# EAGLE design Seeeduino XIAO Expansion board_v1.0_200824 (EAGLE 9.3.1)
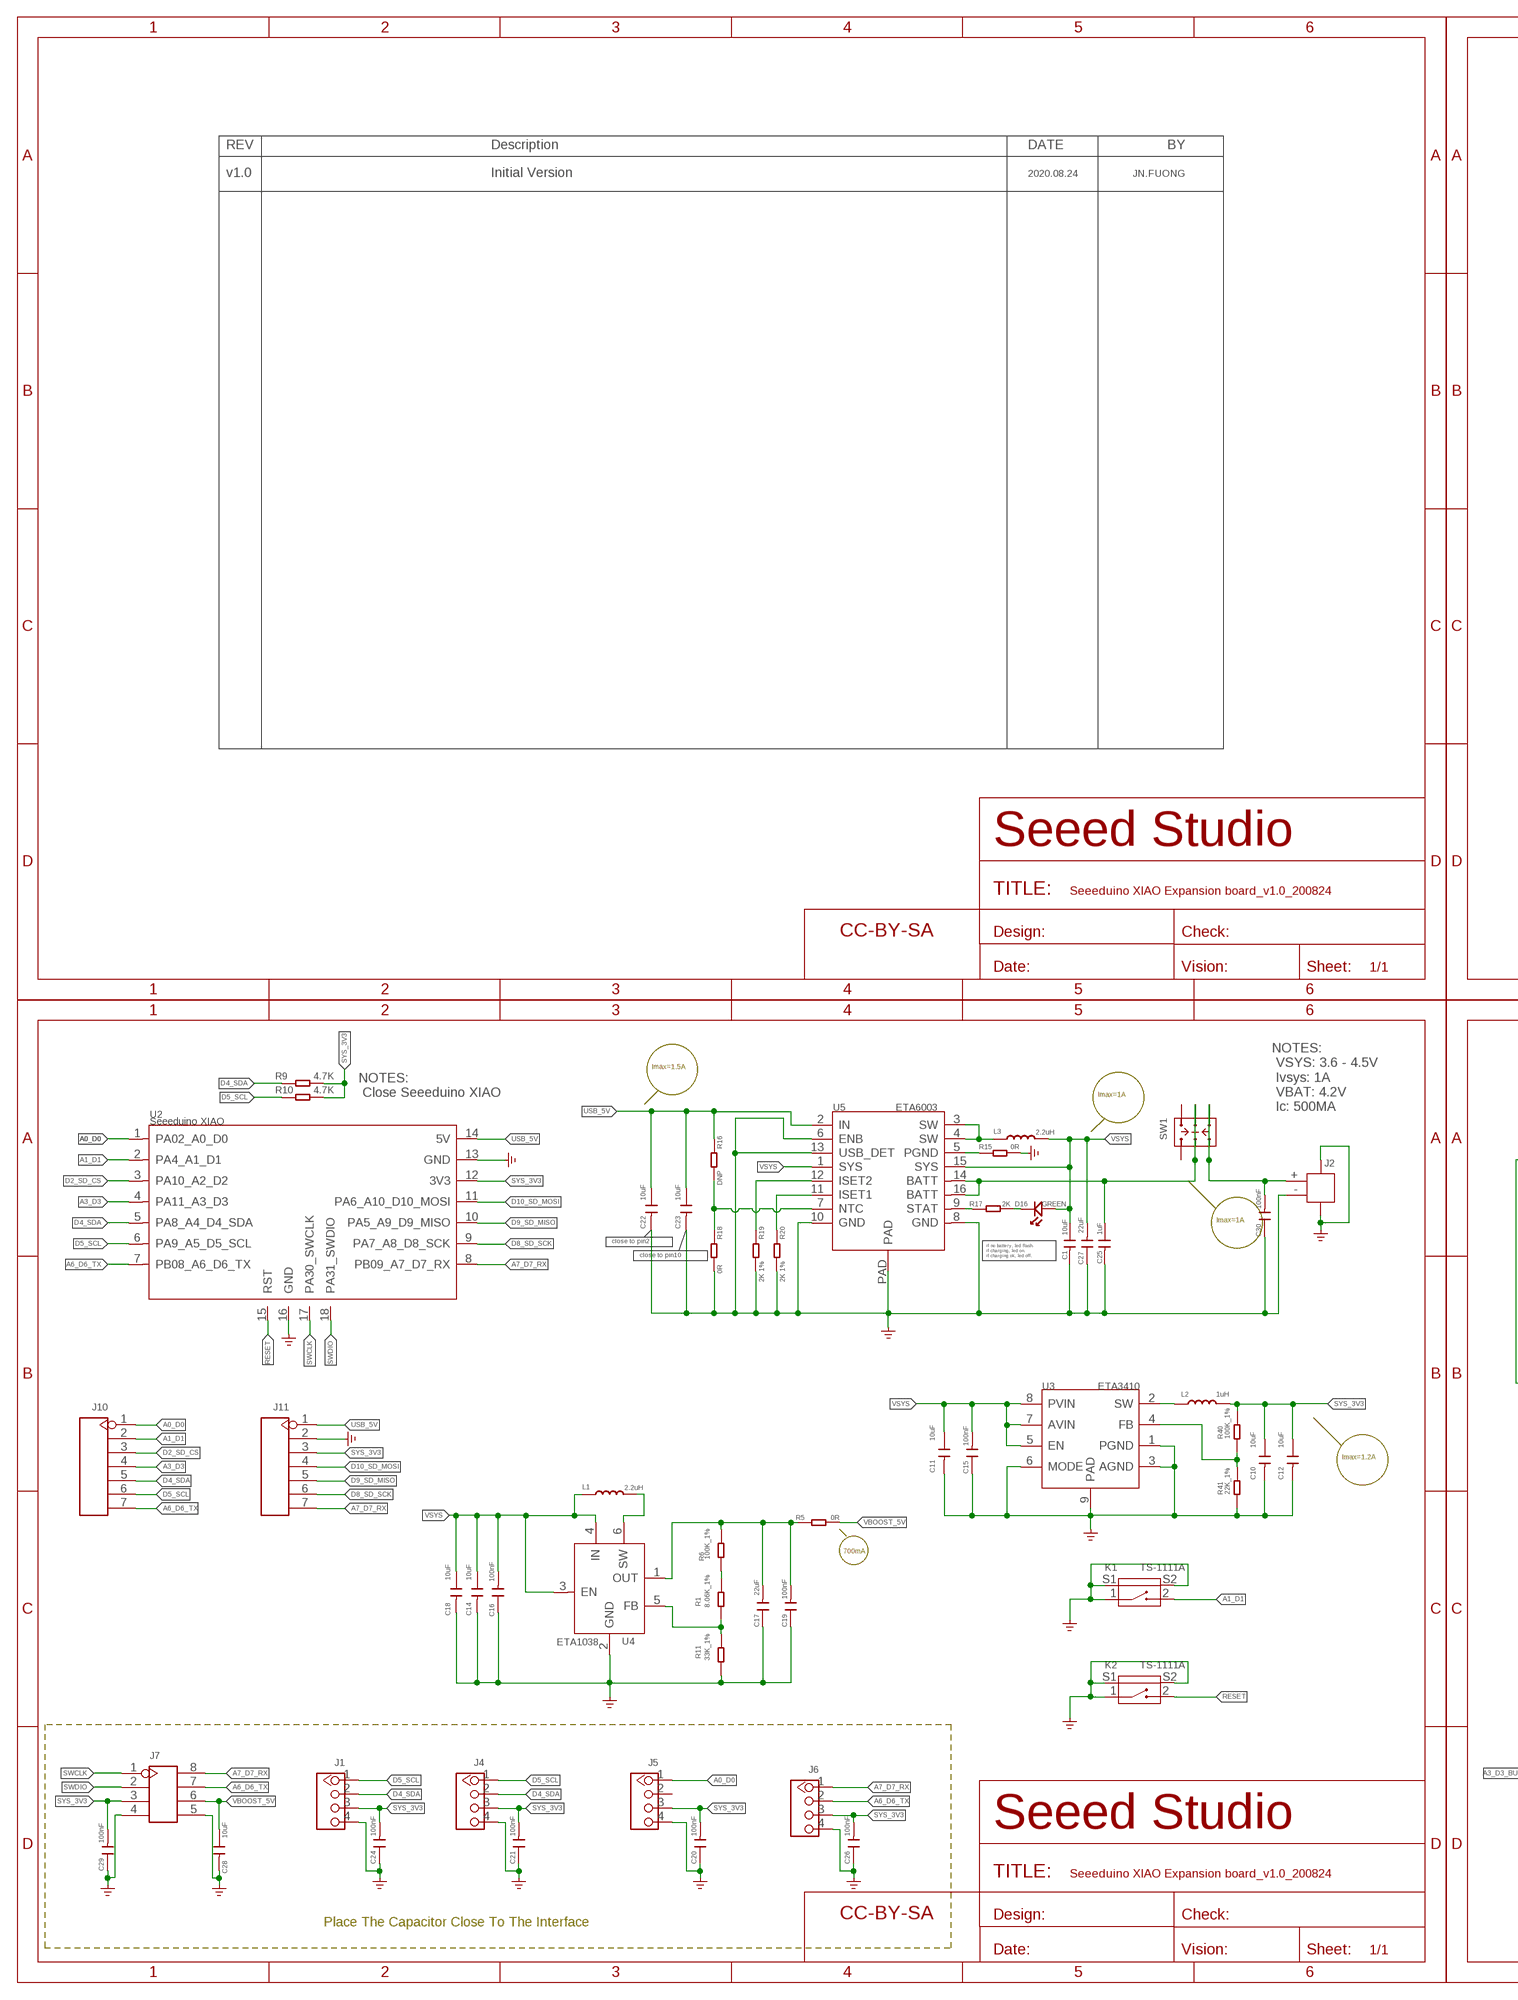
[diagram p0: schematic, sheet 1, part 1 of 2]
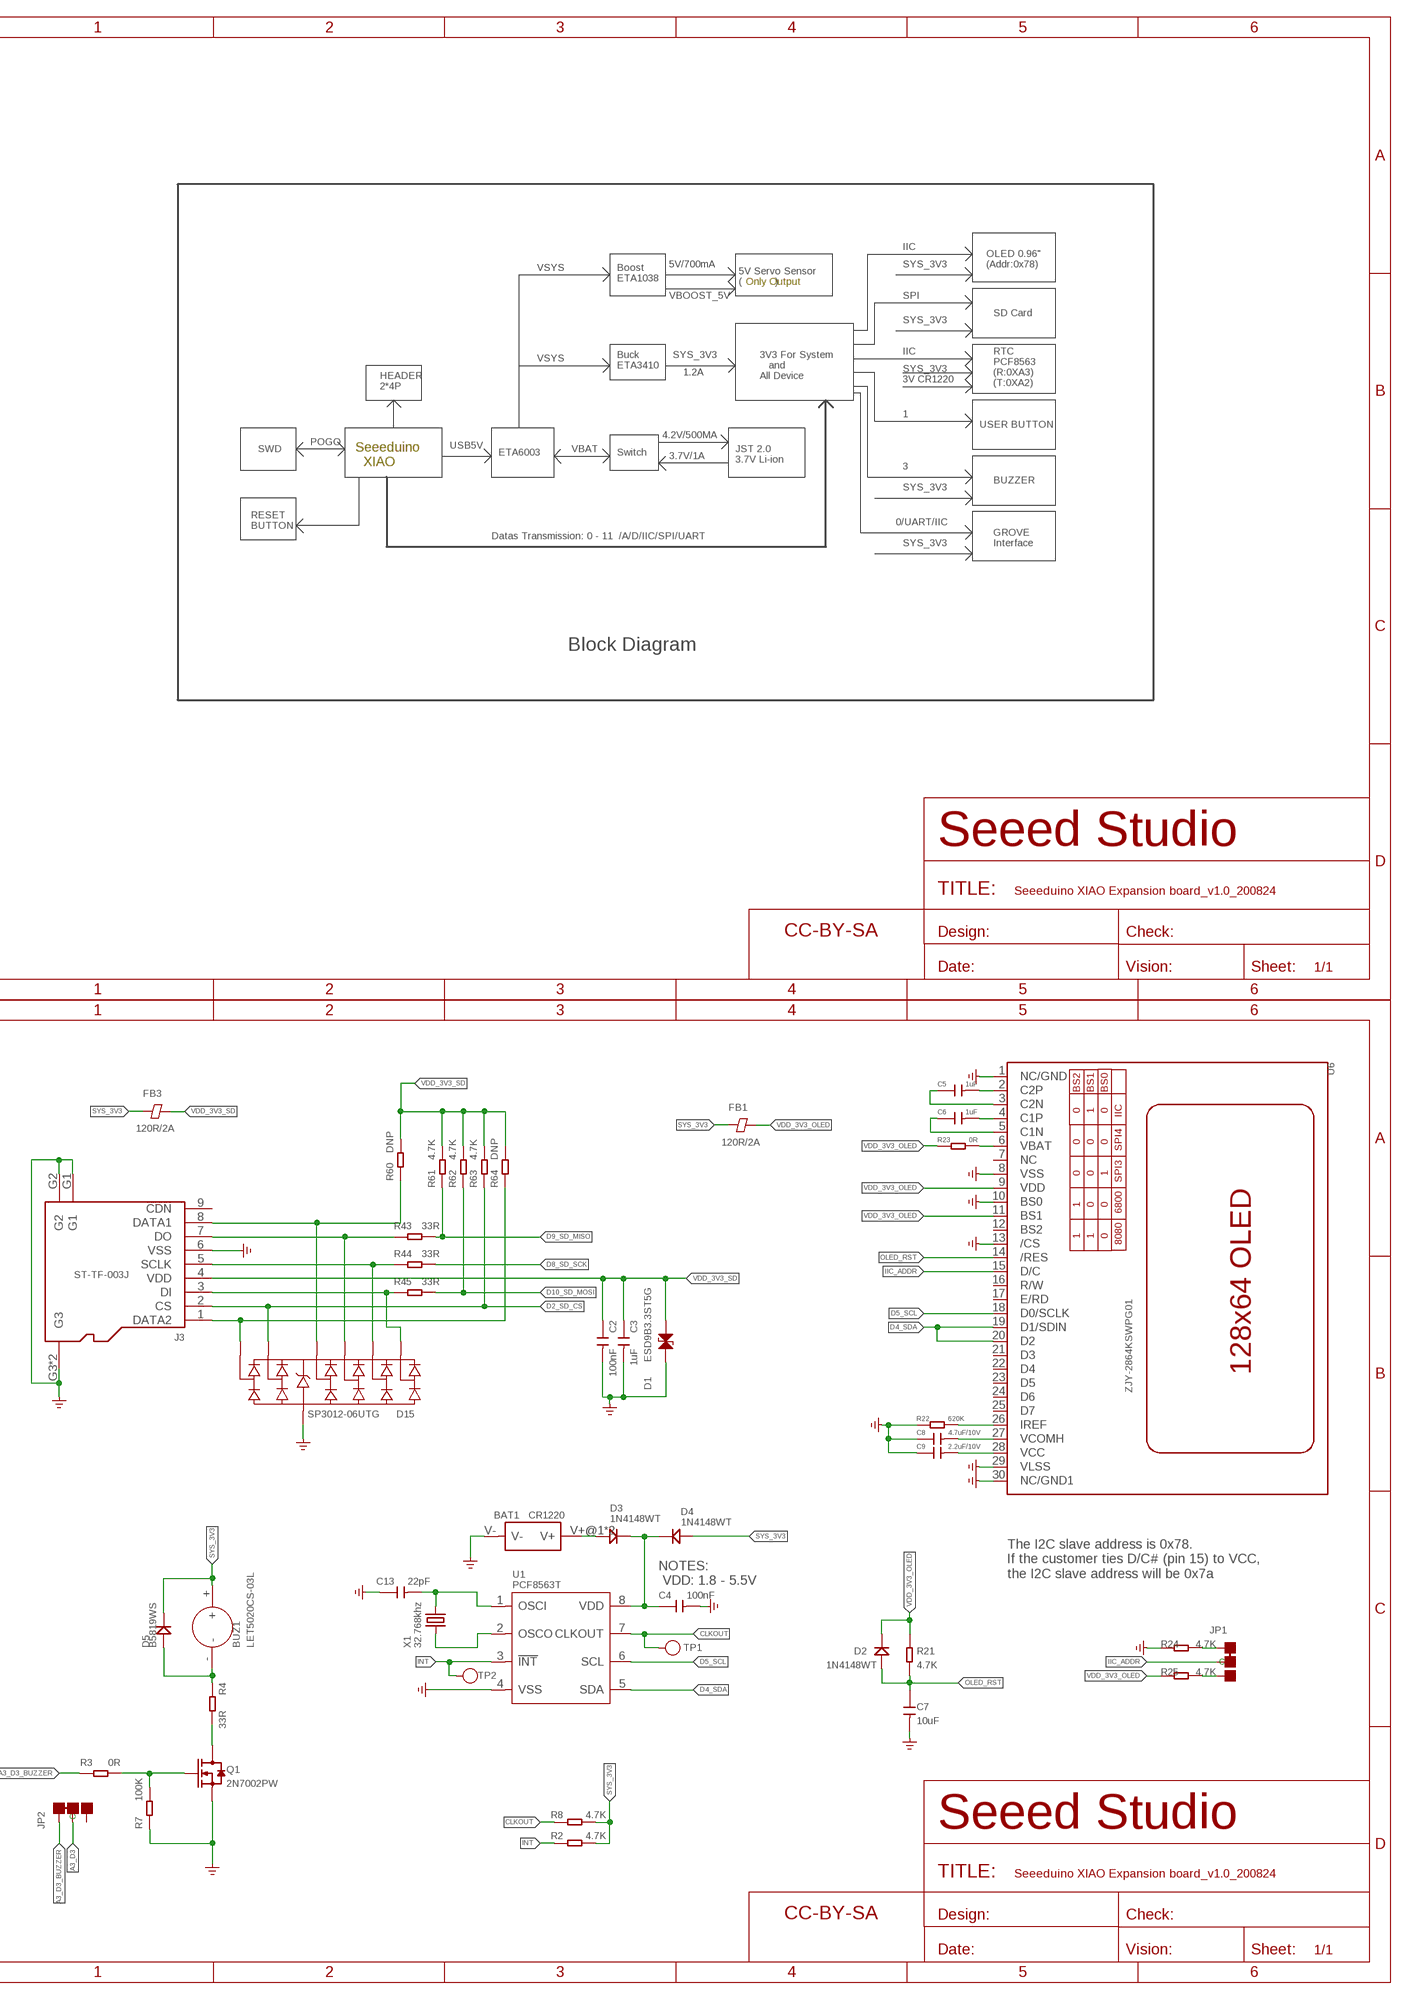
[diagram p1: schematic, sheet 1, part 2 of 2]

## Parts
BAT1  CR1220  BAT-HOLDER-KST-1206  [BAT2P-SMD-13.2X12.1X3.2MM]
BUZ1  LET5020CS-03L  BUZZER-312020004  [BZ3-SMD-5.0X5.0X2.5MM]
C1  10uF  C-0603  [C0603]
C2  100nF  C-0402  [C0402]
C3  1uF  C-0402  [C0402]
C4  100nF  C-0402  [C0402]
C5  1uF  C-0402  [C0402]
C6  1uF  C-0402  [C0402]
C7  10uF  C-0603  [C0603]
C8  4.7uF/10V  C-0603  [C0603]
C9  2.2uF/10V  C-0603  [C0603]
C10  10uF  C-0603  [C0603]
C11  10uF  C-0603  [C0603]
C12  10uF  C-0603  [C0603]
C13  22pF  C-0402  [C0402]
C14  10uF  C-0603  [C0603]
C15  100nF  C-0402  [C0402]
C16  100nF  C-0402  [C0402]
C17  22uF  C-0603  [C0603]
C18  10uF  C-0603  [C0603]
C19  100nF  C-0402  [C0402]
C20  100nF  C-0402  [C0402]
C21  100nF  C-0402  [C0402]
C22  10uF  C-0603  [C0603]
C23  10uF  C-0603  [C0603]
C24  100nF  C-0402  [C0402]
C25  1uF  C-0402  [C0402]
C26  100nF  C-0402  [C0402]
C27  22uF  C-0603  [C0603]
C28  10uF  C-0603  [C0603]
C29  100nF  C-0402  [C0402]
C30  100nF  C-0603  [C0603]
D1  ESD9B3.3ST5G  D-ESD-2P-DOUBLE-0402  [ESD-0402]
D2  1N4148WT  DIODE'0603'  [SOD-523]
D3  1N4148WT  DIODE'0603'  [SOD-523]
D4  1N4148WT  DIODE'0603'  [SOD-523]
D5  B5819WS  DIODE'0805'  [SOD-323]
D15  SP3012-06UTG  D-ESD-14P  [UDFN14-0.5-3.5X1.35X0.5MM]
D16  GREEN  LED-0402  [LED-0402]
FB1  120R/2A  FERRITE-BEAD-0402  [F0402]
FB3  120R/2A  FERRITE-BEAD-0402  [F0402]
FR1  SEEEDSTUDIO-OPEN-SCH-FRAME  [SEEEDSTUDIO-PCB-FRAME]
FR2  SEEEDSTUDIO-OPEN-SCH-FRAME  [SEEEDSTUDIO-PCB-FRAME]
FR3  SEEEDSTUDIO-OPEN-SCH-FRAME  [SEEEDSTUDIO-PCB-FRAME]
FR5  SEEEDSTUDIO-OPEN-SCH-FRAME  [SEEEDSTUDIO-PCB-FRAME]
J1  GROVE-CONNECTOR-DIP-320110034  [HW4-2.0-90D]
J2  JST-2P-SMD'2.0'  [HW2-SMD-2.0-90D]
J3  ST-TF-003J  MICRO-SD-CARD-HOLDER-9P-320090000  [MICRO-SD9+4P-SMD-16.1X14.5X1.85MM]
J4  GROVE-CONNECTOR-DIP-320110034  [HW4-2.0-90D]
J5  GROVE-CONNECTOR-DIP-320110034  [HW4-2.0-90D]
J6  GROVE-CONNECTOR-DIP-320110034  [HW4-2.0-90D]
J7  HEADER-2X4P-2.54-SMD  [H2X4-SMD-2.54]
J10  HEADER-7P-2.54  [H7-2.54]
J11  HEADER-7P-2.54  [H7-2.54]
JP1  JP-3P-SHORT  [3P-SMD-SHORT]
JP2  JP-3P-SHORT  [3P-SMD-SHORT]
K1  TS-1111A  BUTTON-2+2P'HQ-TP-1100A'  [SW4-SMD-4.5X3.8X1.8MM-90D]
K2  TS-1111A  BUTTON-2+2P'HQ-TP-1100A'  [SW4-SMD-4.5X3.8X1.8MM-90D]
L1  2.2uH  INDUCTOR/FERRITE-BEAD'0806'  [L0806]
L2  1uH  L-MPM201610SR33_T  [L201610]
L3  2.2uH  INDUCTOR/FERRITE-BEAD'0806'  [L0806]
Q1  2N7002PW  MOSFET-N-SI1304BDL  [SOT-323]
R1  8.06K_1%  R-0402  [R0402]
R2  4.7K  R-0402  [R0402]
R3  0R  R-0402  [R0402]
R4  33R  R-0402  [R0402]
R5  0R  R-0603  [R0603]
R6  100K_1%  R-0402  [R0402]
R7  100K  R-0402  [R0402]
R8  4.7K  R-0402  [R0402]
R9  4.7K  R-0402  [R0402]
R10  4.7K  R-0402  [R0402]
R11  33K_1%  R-0402  [R0402]
R15  0R  R-0402  [R0402]
R16  DNP  R-0402  [R0402]
R17  2K  R-0402  [R0402]
R18  0R  R-0402  [R0402]
R19  2K 1%  R-0402  [R0402]
R20  2K 1%  R-0402  [R0402]
R21  4.7K  R-0402  [R0402]
R22  620K  R-0402  [R0402]
R23  0R  R-0402  [R0402]
R24  4.7K  R-0402  [R0402]
R25  4.7K  R-0402  [R0402]
R40  100K_1%  R-0402  [R0402]
R41  22K_1%  R-0402  [R0402]
R43  33R  R-0402  [R0402]
R44  33R  R-0402  [R0402]
R45  33R  R-0402  [R0402]
R60  DNP  R-0402  [R0402]
R61  4.7K  R-0402  [R0402]
R62  4.7K  R-0402  [R0402]
R63  4.7K  R-0402  [R0402]
R64  DNP  R-0402  [R0402]
SW1  SWITCH-2CH-6P-311030004  [SW6-2.54-9.0X3.5X3.2MM-90D]
TP1  TEST-POINT'4545'  [TP-D45MIL]
TP2  TEST-POINT'4545'  [TP-D45MIL]
U1  PCF8563T  RTC-PCF8563T  [SOP8-1.27-5X3.9MM]
U2  Seeeduino XIAO  MOUDLE-SEEEDUINO-XIAO-TEST-DIP  [MOUDLE14P-2.54-21X17.8MM-TEST]
U3  ETA3410  CONVERTER-ETA3410  [DFN8G-0.5-2X2MM]
U4  ETA1038  CONVERTER-ETA1038  [SOT-23-6]
U5  ETA6003  PMIC-ETA6003-310990023  [QFN16GA-0.5-3X3MM]
U6  ZJY-2864KSWPG01  OLED-12864-30P  [OLED30P-0.7-24.74X16.9MM]
X1  32.768khz  CRYSTAL-2P'NX2012SA'  [X2-SMD-L2.0X1.2X0.55MM]

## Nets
A0_D0: J5.1 J10.1 U2.1(PA02_A0_D0)
A1_D1: J10.2 K1.2 U2.2(PA4_A1_D1)
A3_D3: J10.4 JP2.MM(C) U2.4(PA11_A3_D3)
A3_D3_BUZZER: JP2.11(L) R3.1
A6_D6_TX: J6.2 J7.7 J10.7 U2.7(PB08_A6_D6_TX)
A7_D7_RX: J6.1 J7.8 J11.7 U2.8(PB09_A7_D7_RX)
CLKOUT: R8.1 TP1.T U1.7(CLKOUT)
D2_SD_CS: D15.6 D15.9 J3.2(CS) J10.3 R63.1 U2.3(PA10_A2_D2)
D4_SDA: J1.2 J4.2 J10.5 R9.1 U1.5(SDA) U2.5(PA8_A4_D4_SDA) U6.19(D1/SDIN) U6.20(D2)
D5_SCL: J1.1 J4.1 J10.6 R10.1 U1.6(SCL) U2.6(PA9_A5_D5_SCL) U6.18(D0/SCLK)
D8_SD_SCK: J11.6 R44.2 U2.9(PA7_A8_D8_SCK)
D9_SD_MISO: J11.5 R43.2 R61.1 U2.10(PA5_A9_D9_MISO)
D10_SD_MOSI: J11.4 R45.2 R62.1 U2.11(PA6_A10_D10_MOSI)
E_VBAT: C30.2 J2.+ SW1.CH1B SW1.CH2B
GND: BAT1.V- C1.2 C2.2 C3.2 C4.2 C7.2 C8.1 C9.1 C10.2 C11.2 C12.2 C13.1 C14.2 C15.1 C16.1 C17.1 C18.2 C19.1 C20.1 C21.1 C22.2 C23.2 C24.1 C25.2 C26.1 C27.1 C28.2 C29.1 C30.1 D1.1 D15.5 D15.10 J1.4 J2.3 J2.4 J2.- J3.6(VSS) J3.G1 J3.G2 J3.G3 J3.G4(G3) J4.4 J5.4 J6.4 J7.4 J7.5 J11.2 K1.1 K1.S1 K1.S2 K2.1 K2.S1 K2.S2 Q1.2(S) R7.1 R11.2 R15.2 R18.2 R19.2 R20.2 R22.2 R24.1 R41.1 U1.4(VSS) U2.13(GND) U2.16(GND) U3.1(PGND) U3.3(AGND) U3.6(MODE) U3.9(PAD) U4.2(GND) U5.6(ENB) U5.8(GND) U5.10(GND) U5.13(USB_DET) U5.PAD U6.1(NC/GND) U6.8(VSS) U6.10(BS0) U6.13(/CS) U6.29(VLSS) U6.30(NC/GND1) ; supply symbol labelled GND_POWER
IIC_ADDR: JP1.MM(C) U6.15(D/C)
INT: R2.1 TP2.T U1.3(!INT)
N$1: L1.2 U4.6(SW)
N$5: BAT1.V+@1(V+) BAT1.V+@2(V+) D3.+
N$6: Q1.3(D) R4.2
N$7: BUZ1.- D5.+ R4.1
N$8: Q1.1(G) R3.2 R7.2
N$9: C5.2 U6.2(C2P)
N$10: C13.2 U1.1(OSCI) X1.2
N$11: U1.2(OSCO) X1.1
N$12: C6.2 U6.4(C1P)
N$13: C5.1 U6.3(C2N)
N$14: C6.1 U6.5(C1N)
N$15: R22.1 U6.26(IREF)
N$16: C8.2 U6.27(VCOMH)
N$17: C9.2 U6.28(VCC)
N$18: R23.2 U6.6(VBAT)
N$19: JP1.11(L) R24.2
N$20: JP1.00(R) R25.2
N$21: R40.1 R41.2 U3.4(FB)
N$22: C17.2 C19.2 R5.2 R6.1 U4.1(OUT)
N$23: C4.1 D3.- D4.- U1.8(VDD)
N$24: R1.1 R6.2
N$26: L3.1 U5.3(SW) U5.4(SW)
N$27: R1.2 R11.1 U4.5(FB)
N$29: L2.1 U3.2(SW)
N$30: D16.- R17.1
N$31: R17.2 U5.9(STAT)
N$33: R16.2 R18.1 U5.7(NTC)
N$34: R20.1 U5.11(ISET1)
N$36: R19.1 U5.12(ISET2)
N$37: R15.1 U5.5(PGND)
N$64: D15.1 D15.14 J3.8(DATA1) R60.1
N$72: D15.7 D15.8 J3.1(DATA2) R64.1
N$76: D15.2 D15.13 J3.7(DO) R43.1
N$77: D15.3 D15.12 J3.5(SCLK) R44.1
N$78: D15.4 D15.11 J3.3(DI) R45.1
OLED_RST: C7.1 D2.+ R21.1 U6.14(/RES)
RESET: K2.2 U2.15(RST)
SWCLK: J7.1 U2.17(PA30_SWCLK)
SWDIO: J7.2 U2.18(PA31_SWDIO)
SYS_3V3: BUZ1.+ C10.1 C12.1 C20.2 C21.2 C24.2 C26.2 C29.2 D4.+ D5.- FB1.1 FB3.1 J1.3 J4.3 J5.3 J6.3 J7.3 J11.3 L2.2 R2.2 R8.2 R9.2 R10.2 R40.2 U2.12(3V3)
USB_5V: C22.1 C23.1 J11.1 R16.1 U2.14(5V) U5.2(IN)
VBAT: C25.1 SW1.COM1 SW1.COM2 U5.14(BATT) U5.16(BATT)
VBOOST_5V: C28.1 J7.6 R5.1
VDD_3V3_OLED: D2.- FB1.2 R21.2 R23.1 R25.1 U6.9(VDD) U6.11(BS1)
VDD_3V3_SD: C2.1 C3.1 D1.2 FB3.2 J3.4(VDD) R60.2 R61.2 R62.2 R63.2 R64.2
VSYS: C1.1 C11.1 C14.1 C15.2 C16.2 C18.1 C27.2 D16.+ L1.1 L3.2 U3.5(EN) U3.7(AVIN) U3.8(PVIN) U4.3(EN) U4.4(IN) U5.1(SYS) U5.15(SYS)
Unconnected: J3.9(CDN) J5.2 JP2.00(R) SW1.CH1A SW1.CH2A U6.7(NC) U6.12(BS2) U6.16(R/W) U6.17(E/RD) U6.21(D3) U6.22(D4) U6.23(D5) U6.24(D6) U6.25(D7)

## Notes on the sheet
- v1.0 | Initial Version | 2020.08.24 | JN.FUONG
- IIC
- VSYS
- 5V/700mA | SYS_3V3
- OLED 0.96"
  (Addr:0x78)
- Boost
  ETA1038
- 5V Servo Sensor
  (           )
- Only Output
- VBOOST_5V | SPI
- SD Card
- SYS_3V3
- VSYS | IIC
- SYS_3V3
- Buck
  ETA3410
- SYS_3V3
- 1.2A
- 3V3 For System 
     and 
  All Device
- 3V CR1220
- RTC
  PCF8563
  (R:0XA3)
  (T:0XA2)
- HEADER
  2*4P
- 1
- USER BUTTON
- 4.2V/500MA
- POGO
- USB5V
- SWD | VBAT
- ETA6003 | Switch
- 3.7V/1A
- JST 2.0
  3.7V Li-ion
- Seeeduino
    XIAO
- 3
- BUZZER
- SYS_3V3
- 0/UART/IIC
- RESET
  BUTTON
- Datas Transmission: 0 - 11  /A/D/IIC/SPI/UART
- SYS_3V3
- GROVE 
  Interface
- Block Diagram
- Imax=1.5A
- NOTES:
   Close Seeeduino XIAO
- Imax=1A
- NOTES:
   VSYS: 3.6 - 4.5V
   Ivsys: 1A
   VBAT: 4.2V
   Ic: 500MA
- Imax=1A
- close to pin2
- close to pin10
- if no battery, led flash.
  if charging, led on.
  if charging ok, led off.
- Imax=1.2A
- 700mA
- The I2C slave address is 0x78.
  If the customer ties D/C# (pin 15) to VCC,
  the I2C slave address will be 0x7a
- NOTES:
   VDD: 1.8 - 5.5V
- Place The Capacitor Close To The Interface

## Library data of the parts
BAT1 = Connector-new:BAT-HOLDER: BAT2P-13.5-CR1220:320170002;BAT2P-SMD-20.5-CR1632:320170007;METAL-CR2032-D20.0*H6.3MM:320170003;METAL-CR2032-SMD:320170006;PLASTIC-CR1220-L15.06*W13.0*H4.1MM:32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
BUZ1 = Discrete-new:BUZZER
C1-C30 = Discrete-small:C*: Ceramic Capacitors
D1 = Discrete-small:D-ESD-2P-DOUBLE
D2-D5 = Discrete-new:DIODE
D15 = Discrete-new:D-ESD-14P
D16 = Discrete-small:LED
FB1 FB3 = Discrete-new:FERRITE-BEAD
FR1-FR3 FR5 = moudle-new:SEEEDSTUDIO-OPEN-SCH-FRAME
J1 J4-J6 = Connector-new:GROVE-CONNECTOR-DIP
J2 = Connector-new:JST-2P-SMD
J3 = Connector-new:MICRO-SD-CARD-HOLDER-9P; SKU: 320090000
J7 = Connector-new:HEADER-2X4P
J10 J11 = Connector-new:HEADER-7P
JP1 JP2 = Discrete-new:JP-3P-SHORT
K1 K2 = Discrete-new:BUTTON-2+2P: SW4-SMD-4.5X3.8X1.8MM-90D:311020035;SW4-SMD-7.0X3.5X3.5MM-90D:311020023
L1 L3 = Discrete-new:INDUCTOR/FERRITE-BEAD
L2 = Discrete-new:L
Q1 = Discrete-new:MOSFET-N: IRLL014: http://www.vishay.com/docs/91319/sihll014.pdf
R1-R11 R15-R25 R40 R41 R43-R45 R60-R64 = Discrete-small:R*
SW1 = Switch:SWITCH-2CH-6P
TP1 TP2 = Discrete-new:TEST-POINT; PARTNO: DNP
U1 = IC-new:RTC-PCF8563T
U2 = moudle-new:MOUDLE-SEEEDUINO-XIAO-TEST
U3 = IC-new:CONVERTER-ETA3410: 3MHZ 2A High Step-Down Converter in DFN2x2-8L Package
U4 = IC-new:CONVERTER-ETA1038
U5 = IC-new:PMIC-ETA6003
U6 = moudle-new:OLED-128*64-30P: 308020008
X1 = Discrete-new:CRYSTAL-2P

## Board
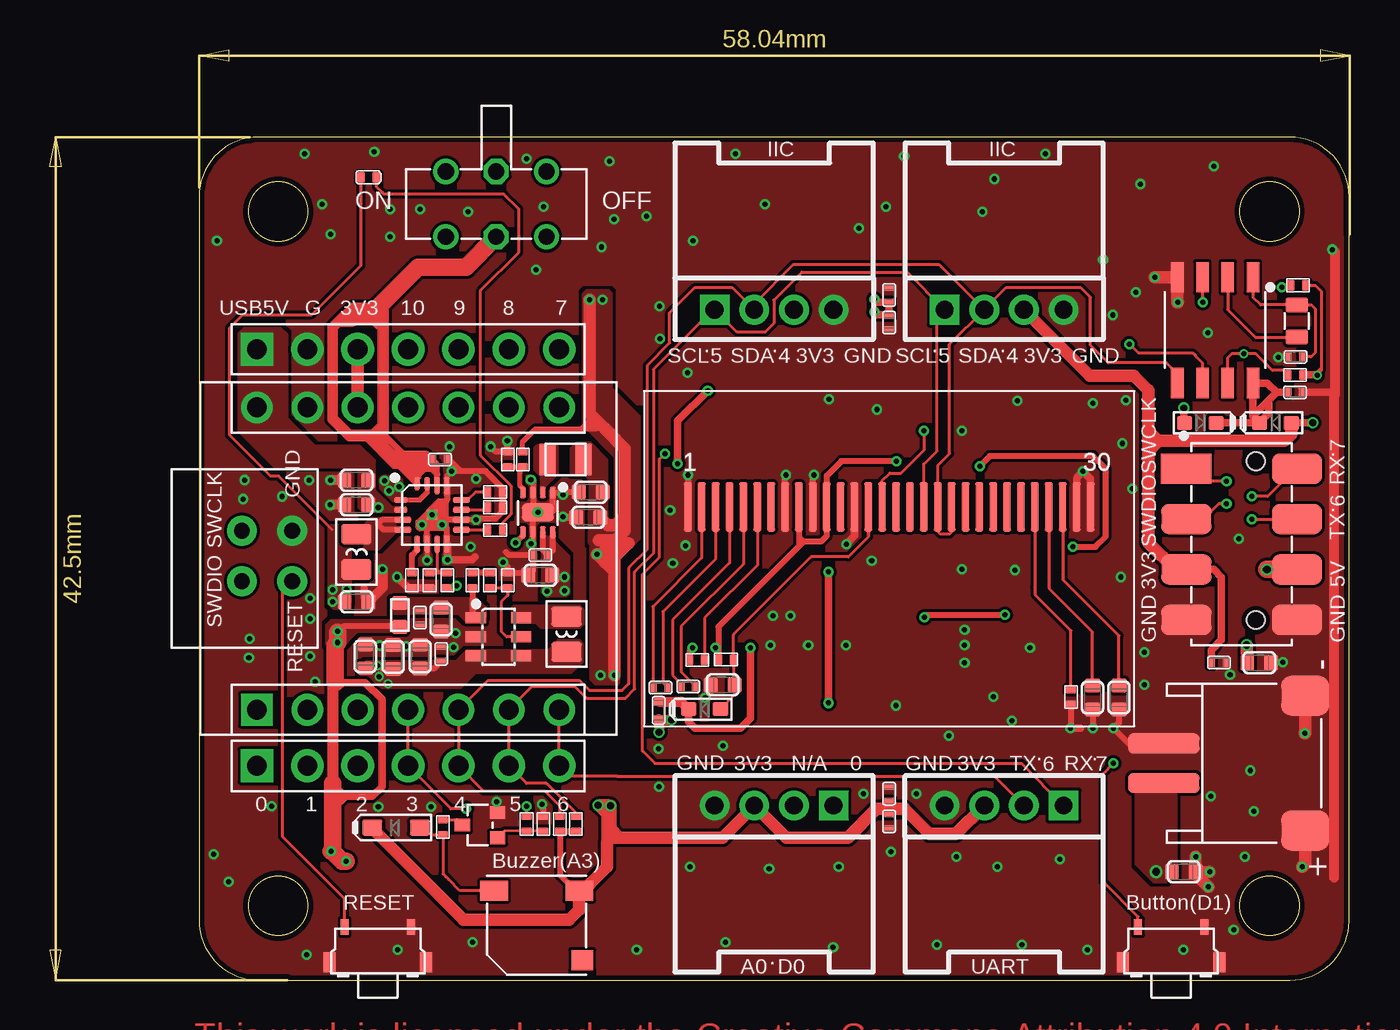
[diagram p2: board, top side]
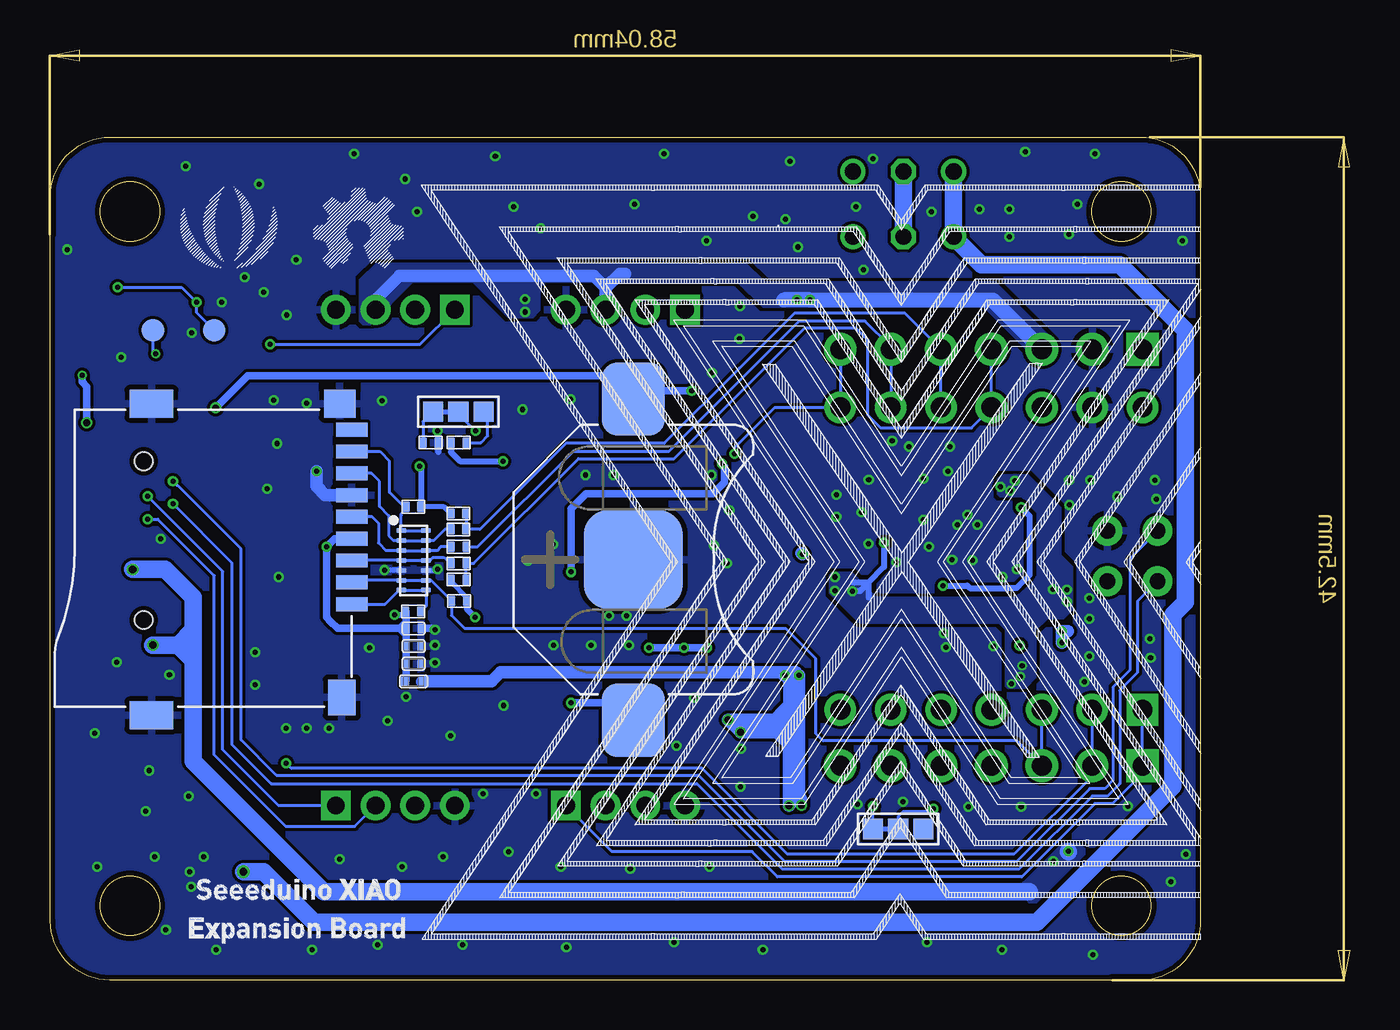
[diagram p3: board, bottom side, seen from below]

Size 65.58 x 46.91 mm. Coordinates in mm from the lower left corner, seen from the top.
Outline: 62.54,42.5 10.54,42.5 arc90 7.54,39.5 7.54,3 arc90 10.54,0 62.54,0 arc90 65.54,3 65.54,39.5 arc90 62.54,42.5
Outline: circle at 11.53,38.75 radius 1.5
Outline: circle at 61.53,38.75 radius 1.5
Outline: circle at 61.53,3.75 radius 1.5
Outline: circle at 11.53,3.75 radius 1.5
Copper layers (1*16): Top 0.035mm / dielectric 1.5mm / Bottom 0.035mm
Design rules "SeeedStudio_2layer_DRU_no_angle_20140221": minimum track width 1mil, minimum drill 10mil, track to track 6mil, track to pad 6mil, pad to pad 6mil, via to via 6mil, smd to smd 0mil, copper to edge 10mil, drill to drill 10mil, minimum pad ring 4mil, minimum via ring 4mil, stop-mask expansion 2mil, vias tented up to drill 25mil, thermal gap 10mil

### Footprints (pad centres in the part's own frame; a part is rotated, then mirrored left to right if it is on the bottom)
BAT2P-SMD-13.2X12.1X3.2MM = smd 3.7 x 3.2: V+@1 -8.1,0; V+@2 8.1,0 | smd 5 x 5: V- 0,0
BZ3-SMD-5.0X5.0X2.5MM = smd 1.4 x 1: + -2.15,-1.75; - 2.15,-1.75 | smd 1.1 x 1: NC -2.3,1.75
C0603 = smd 0.762 x 0.696: 1 0,0.602; 2 0,-0.602
C0402 = smd 0.508 x 0.385: 1 0,0.383; 2 0,-0.383
ESD-0402 = smd 0.385 x 0.508: 1 0.383,0; 2 -0.383,0
SOD-523 = smd 0.762 x 0.7: + 0.8,0; - -0.8,0
SOD-323 = smd 1 x 0.8: + 1.2,0; - -1.2,0
UDFN14-0.5-3.5X1.35X0.5MM = smd 0.25 x 0.5: 1 -1.5,-0.625; 2 -1,-0.625; 3 -0.5,-0.625; 4 0,-0.625; 5 0.5,-0.625; 6 1,-0.625; 7 1.5,-0.625; 8 1.5,0.625; 9 1,0.625; 10 0.5,0.625; 11 0,0.625; 12 -0.5,0.625; 13 -1,0.625; 14 -1.5,0.625
LED-0402 = smd 0.385 x 0.508: + -0.383,0; - 0.383,0
F0402 = smd 0.445 x 0.508: 1 -0.445,0; 2 0.445,0
HW4-2.0-90D = drill 0.9 pad 1.5 square: 1 -3,0 | drill 0.9 pad 1.5: 2 -1,0; 3 1,0; 4 3,0
HW2-SMD-2.0-90D = smd 2 x 2.4: 3 3.4,-2.181; 4 -3.4,-2.181 | smd 1 x 3.6: + -1,4.953; - 1,4.953
MICRO-SD9+4P-SMD-16.1X14.5X1.85MM = smd 1.6 x 0.7: 1 0,2.25; 2 0,1.15; 3 0,0.05; 4 0,-1.05; 5 0,-2.15; 6 0,-3.25; 7 0,-4.35; 8 0,-5.45; 9 0,-6.55 | smd 1.6 x 1.4: G1 0.6,-7.85 | smd 2.2 x 1.4: G2 10.1,-7.85; G3 10.1,7.85 | smd 1.4 x 1.8: G4 0.5,6.95 | hole 0.9: 10.5,-4.95; 10.5,3.05
H2X4-SMD-2.54 = smd 2.54 x 1.524: 1 -2.794,3.81; 2 -2.794,1.27; 3 -2.794,-1.27; 4 -2.794,-3.81; 5 2.794,-3.81; 6 2.794,-1.27; 7 2.794,1.27; 8 2.794,3.81
H7-2.54 = drill 1 pad 1.651 square: 1 0,7.62 | drill 1 pad 1.651: 2 0,5.08; 3 0,2.54; 4 0,0; 5 0,-2.54; 6 0,-5.08; 7 0,-7.62
3P-SMD-SHORT = smd 1.016 x 1.016: 00 -1.27,0; 11 1.27,0; MM 0,0
SW4-SMD-4.5X3.8X1.8MM-90D = smd 0.4 x 0.8: 1 -1.675,-1.277; 2 1.675,-1.277 | smd 0.6 x 1: S1 -2.425,0.5; S2 2.425,0.5
L0806 = smd 1.016 x 1.524: 1 -0.889,0; 2 0.889,0
L201610 = smd 0.8 x 1.6: 1 -0.9,0; 2 0.9,0
SOT-323 = smd 0.762 x 0.635: 1 0.889,-0.635; 2 0.889,0.635; 3 -0.889,0
R0402 = smd 0.385 x 0.508: 1 0.383,0; 2 -0.383,0
R0603 = smd 0.696 x 0.762: 1 0.602,0; 2 -0.602,0
SW6-2.54-9.0X3.5X3.2MM-90D = drill 0.813 pad 1.27: CH1A -2.54,-1.65; CH1B 2.54,-1.65; CH2A -2.54,1.65; CH2B 2.54,1.65 | drill 0.813 pad 1.27 octagon: COM1 0,-1.65; COM2 0,1.65
TP-D45MIL = smd 1.143 x 1.143: T 0,0
SOP8-1.27-5X3.9MM = smd 0.635 x 1.524: 1 -1.905,-2.667; 2 -0.635,-2.667; 3 0.635,-2.667; 4 1.905,-2.667; 5 1.905,2.667; 6 0.635,2.667; 7 -0.635,2.667; 8 -1.905,2.667
MOUDLE14P-2.54-21X17.8MM-TEST = drill 1 pad 1.6 square: 1 7.62,7.62 | drill 1 pad 1.6: 2 5.08,7.62; 3 2.54,7.62; 4 0,7.62; 5 -2.54,7.62; 6 -5.08,7.62; 7 -7.62,7.62; 8 -7.62,-7.62; 9 -5.08,-7.62; 10 -2.54,-7.62; 11 0,-7.62; 12 2.54,-7.62; 13 5.08,-7.62; 14 7.62,-7.62 | drill 0.8 pad 1.5: 15 5.842,1.143; 16 5.842,-1.397; 17 8.382,-1.397; 18 8.382,1.143
DFN8G-0.5-2X2MM = smd 0.3 x 0.6: 1 -0.75,-1; 2 -0.25,-1; 3 0.25,-1; 4 0.75,-1; 5 0.75,1; 6 0.25,1; 7 -0.25,1; 8 -0.75,1 | smd 1.6 x 0.9: 9 0,0
SOT-23-6 = smd 0.55 x 1.016: 1 -0.95,-1.143; 2 0,-1.143; 3 0.95,-1.143; 4 0.95,1.143; 5 0,1.143; 6 -0.95,1.143
QFN16GA-0.5-3X3MM = smd 0.28 x 0.65: 1 -0.75,-1.575; 2 -0.25,-1.575 | smd 0.28 x 0.85: 3 0.25,-1.475; 4 0.75,-1.475; 9 0.75,1.475; 10 0.25,1.475; 11 -0.25,1.475; 12 -0.75,1.475 | smd 0.85 x 0.28: 5 1.475,-0.75; 6 1.475,-0.25; 7 1.475,0.25; 8 1.475,0.75; 13 -1.475,0.75; 14 -1.475,0.25 | smd 0.65 x 0.28: 15 -1.575,-0.25; 16 -1.575,-0.75 | smd 0.508 x 0.508: PAD 0,0
OLED30P-0.7-24.74X16.9MM = smd 0.4 x 2.5: 1 -10.15,2.604; 2 -9.45,2.604; 3 -8.75,2.604; 4 -8.05,2.604; 5 -7.35,2.604; 6 -6.65,2.604; 7 -5.95,2.604; 8 -5.25,2.604; 9 -4.55,2.604; 10 -3.85,2.604; 11 -3.15,2.604; 12 -2.45,2.604; 13 -1.75,2.604; 14 -1.05,2.604; 15 -0.35,2.604; 16 0.35,2.604; 17 1.05,2.604; 18 1.75,2.604; 19 2.45,2.604; 20 3.15,2.604; 21 3.85,2.604; 22 4.55,2.604; 23 5.25,2.604; 24 5.95,2.604; 25 6.65,2.604; 26 7.35,2.604; 27 8.05,2.604; 28 8.75,2.604; 29 9.45,2.604; 30 10.15,2.604
X2-SMD-L2.0X1.2X0.55MM = smd 0.762 x 1.143: 1 -0.813,0; 2 0.813,0

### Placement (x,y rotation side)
BAT1  36.14,21.2 270 bottom
BUZ1  24.56,2.76 180 top
C1  15.48,19.07 90 top
C2  47.22,16.84 90 bottom
C3  47.22,15.95 90 bottom
C4  62.81,29.63 90 top
C5  30.81,14.74 270 top
C6  32.21,14.8 270 top
C7  33.95,14.88 270 top
C8  52.6,14.24 180 top
C9  53.93,14.24 180 top
C10  27.16,23.33 270 top
C11  24.75,20.41 270 top
C12  27.29,24.6 270 top
C13  62.83,31.42 90 top
C14  17.33,16.29 180 top
C15  24.75,21.42 90 top
C16  19.75,16.44 0 top
C17  19.75,18.18 180 top
C18  18.69,16.31 180 top
C19  18.68,18.27 180 top
C20  42.34,34.54 0 top
C21  42.34,33.15 180 top
C22  15.48,25.19 270 top
C23  15.48,23.96 270 top
C24  42.34,8 180 top
C25  19.69,26.25 90 top
C26  42.34,9.4 0 top
C27  15.92,16.32 0 top
C28  61.01,16 90 top
C29  58.97,16 270 top
C30  57.2,5.46 270 top
D1  47.22,17.73 0 bottom
D2  33.03,13.66 0 top
D3  58.03,28.09 180 top
D4  61.82,28.09 0 top
D5  17.48,7.69 0 top
D15  47.22,21.16 270 bottom
D16  16.09,40.47 0 top
FB1  30.71,13.6 90 top
FB3  47.22,15.06 180 bottom
FR1  not placed on the board
FR2  not placed on the board
FR3  not placed on the board
FR5  not placed on the board
J1  48.14,33.8 0 top
J2  61.14,10.94 90 top
J3  50.34,21.2 180 bottom
J4  36.54,33.8 0 top
J5  36.54,8.8 180 top
J6  48.14,8.8 180 top
J7  60.12,21.97 0 top
J10  18.08,10.8 90 top
J11  18.08,31.8 90 top
JP1  44.97,28.66 180 bottom
JP2  22.78,7.62 180 bottom
K1  56.56,1.4 180 top
K2  16.55,1.4 180 top
L1  26.07,17.44 90 top
L2  26.02,26.25 0 top
L3  15.48,21.59 270 top
Q1  21.7,7.81 0 top
R1  22.21,20.15 90 top
R2  62.97,35.03 180 top
R3  24.05,7.87 90 top
R4  19.84,7.71 270 top
R5  17.66,18.4 270 top
R6  21.32,20.15 270 top
R7  24.89,7.87 90 top
R8  62.82,30.51 180 top
R9  25.73,7.87 90 top
R10  26.55,7.87 90 top
R11  23.1,20.15 270 top
R15  18.27,20.15 90 top
R16  20.05,20.15 270 top
R17  22.46,22.69 0 top
R18  19.16,20.15 90 top
R19  22.46,24.6 180 top
R20  22.46,23.84 180 top
R21  34.11,16.15 0 top
R22  51.51,14.27 90 top
R23  32.66,16.14 180 top
R24  46.36,27.09 0 bottom
R25  44.95,27.09 180 bottom
R40  23.86,26.25 270 top
R41  23.1,26.25 90 top
R43  44.97,22.73 180 bottom
R44  44.96,21.85 180 bottom
R45  44.95,21.01 180 bottom
R60  47.23,23.86 180 bottom
R61  44.96,23.52 0 bottom
R62  44.95,20.19 0 bottom
R63  44.93,19.11 180 bottom
R64  47.24,18.58 0 bottom
SW1  22.52,39.12 180 top
TP1  60.37,32.77 270 bottom
TP2  57.29,32.77 90 bottom
U1  58.78,32.77 180 top
U2  18.08,21.25 180 top
U3  24.62,23.58 180 top
U4  22.64,17.31 270 top
U5  19.29,23.45 270 top
U6  42.34,21.25 0 top
X1  62.89,33.22 90 top

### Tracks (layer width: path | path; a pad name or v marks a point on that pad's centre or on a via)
A0_D0
  Bottom 0.152: U2.1 J10.1 10.46,10.41 11.98,8.89 12.87,8.89 16.56,5.21 28.88,5.21 30.15,6.48 37.22,6.48 J5.1
A1_D1  (via drill 0.25 pad 0.51)
  Top 0.152: K1.2 54.89,3.2 53.13,4.95 53.13,10.41 v53.64,10.92
  Bottom 0.152: U2.2 J10.2 13,10.29 16.94,6.35 28.37,6.35 32.69,10.67 53.39,10.67 v53.64,10.92
A3_D3  (via drill 0.25 pad 0.51)
  Top 0.152: U2.4 J10.4 20.24,8.64 v21,8.64
  Bottom 0.152: JP2.MM 22.78,8.26 22.52,8.51 21.13,8.51 v21,8.64
A3_D3_BUZZER  (via drill 0.25 pad 0.51)
  Top 0.152: v24.05,8.76 R3.1
  Bottom 0.152: JP2.11 v24.05,8.76
A6_D6_TX  (via drill 0.25 pad 0.51)
  Top 0.152: U2.7 J10.7 26.21,10.29 28.62,10.29 47.65,10.29 J6.2 | v60.62,23.24 J7.7
  Bottom 0.152: v60.62,23.24 60.12,23.24 57.27,20.4 57.27,11.35 53.66,7.75 50.19,7.75 J6.2
A7_D7_RX  (via drill 0.25 pad 0.51)
  Top 0.152: v31.03,26.54 30.76,26.26 30.76,21.31 29.89,20.45 29.89,11.56 30.53,10.92 49.02,10.92 J6.1 | J7.8 62.83,25.78 61.43,24.38 v60.62,24.38
  Bottom 0.152: v31.03,26.54 31.03,26.84 29,28.87 U2.8 J11.7 | v60.62,24.38 56.84,20.6 56.84,11.61 54.03,8.8 J6.1
CLKOUT  (via drill 0.25)
  Top 0.152: R8.1 62.2,30.73 61.67,30.73 60.84,31.57 v60.23,31.57 v60.22,31.57 59.62,31.57 59.41,31.37 U1.7
  Bottom 0.152: TP1.T 60.37,31.72 v60.22,31.57
D2_SD_CS
  Bottom 0.152: J3.2 50.23,20.16 D15.6 D15.9 46.35,20.16 R63.1 45.31,18.39 44.65,17.73 28.46,17.73 26.95,16.22 26.95,12.45 26.56,12.06 16.8,12.06 J10.3 U2.3
D4_SDA
  Top 0.152: U2.5 J10.5 21.89,9.53 24.99,9.53 25.73,8.78 R9.1 | J1.2 45.38,32.05 45.38,26.54 44.79,25.95 U6.19 44.84,23.8 44.84,22.57 44.93,22.48 45.38,22.48 45.49,22.58 U6.20 | J1.2 44.87,36.07 37.5,36.07 35.54,34.1 J4.2 34.41,34.92 32.56,34.92 31.27,33.64 31.27,32.12 30.15,30.99 30.15,21.72 29.2,20.78 29.2,14.94 28.88,14.61 27.22,14.61 26.72,15.11 22.1,15.11 U2.5 | U2.5 | J1.2 48.26,34.92 51.99,34.92 52.5,34.42 52.5,32 53.39,31.11 56.31,31.11 56.87,30.55 U1.5
D5_SCL  (via drill 0.25 pad 0.51)
  Top 0.152: U1.6 58.14,31.11 57.86,31.4 57.77,31.49 57.63,31.62 54.91,31.62 54.49,32.05 v54.44,32.05 | U6.18 44.09,26.01 44.75,26.67 44.75,33.41 J1.1 43.25,35.69 37.94,35.69 36.53,34.28 36.53,33.11 36.09,32.67 34.67,32.67 J4.1 33.46,33.8 30.45,30.79 30.45,21.51 29.51,20.57 29.51,14.68 29.04,14.21 27.08,14.21 26.51,14.79 24.32,14.79 U2.6 J10.6 24.05,9.91 25.06,9.91 26.55,8.42 R10.1
  Bottom 0.152: v54.44,32.05 46.89,32.05 J1.1
D8_SD_SCK
  Bottom 0.152: R44.2 43.99,21.85 39.16,26.67 34.34,26.67 27.78,33.22 24.45,33.22 23.16,31.93 J11.6 U2.9
D9_SD_MISO
  Bottom 0.152: 30.79,30.85 34.59,27.05 39.54,27.05 43.87,22.73 R43.2 R61.1 | 30.79,30.85 28.02,33.62 22.44,33.62 J11.5 U2.10 | 30.79,30.85
D10_SD_MOSI
  Bottom 0.152: J11.4 U2.11 18.08,28.84 19.09,27.84 23.67,27.84 24.3,28.47 24.3,32.26 24.91,32.87 27.5,32.87 34.08,26.29 38.91,26.29 44.19,21.01 R45.2 R62.1
E_VBAT  (via drill 0.38 pad 0.64)
  Bottom 0.889: v55.8,5.46 54.78,5.46 52.24,2.92 15.79,2.92 8.94,9.78 8.94,18.41 8.3,19.05 8.3,32.77 11.6,36.07 18.59,36.07 SW1.CH2B SW1.CH1B
  pour Top (isolate 0.254, no thermals): 55.93,10.16 55.29,10.16 54.78,9.65 54.78,5.84 55.67,4.95 56.31,4.95 56.82,5.46 56.82,9.65 56.31,10.16
GND  (via drill 0.25 pad 0.51)
  Top 0.152: v19.04,21.18 v19.04,21.17
  Top 0.254: U5.13 20.04,25.43 v20.26,25.65 | U5.10 20.78,23.22 21.48,23.22 | R15.2 | U5.6 v19.04,21.18 | U3.6 24.37,22.09 v24.28,22 24.37,21.91 C15.1
  Top 0.305: 21.48,23.22 21.53,23.27 22.48,23.27 22.85,23.63 R20.2 R19.2 22.85,24.8 21.99,25.65 20.72,25.65 | 20.72,25.65 v20.26,25.65 20.26,26.11 20.72,25.65 | v24.27,25.23 24.37,25.12 U3.3 24.37,23.33 | U3.1 26.02,24.58 | 26.02,24.58 v25.9,24.46 25.78,24.58 U3.1 | C12.2 26.67,24.58 26.02,24.58 | v23.08,27.18 23.1,27.16 R41.1 23.08,26.64 22.5,26.64 v22.25,26.9 | v22.88,21.06 23.1,20.84 R11.2 24.02,20.54 C11.2 24.37,20.63 C15.1 23.17,21.42 23.01,21.59 | C7.2 33.35,14.5 v33.07,14.22 | U6.1 32.19,23.86 v32.19,25.46 | U6.8 37.1,25.42 v37.14,25.46 | U6.10 38.5,25.42 v38.54,25.46 | C9.1 53.93,12.99 v53.64,12.7 54.4,11.94 J2.- | C8.1 52.62,13.62 v52.62,12.7 | v51.48,12.7 51.51,12.7 R22.2 | C13.1 62,31.42 v61.97,31.39 | U3.6 24.37,23.33 | 24.37,23.33 U3.9 | U3.1 25.37,23.65 25.22,23.5 25.24,23.47 | U5.6 19.04,23.2 19.19,23.35 | 19.19,23.35 U5.PAD 20.04,24.2 20.04,24.43 U5.13 | U5.10 19.63,23.2 | 19.63,23.2 19.34,23.2 19.19,23.35 | U5.8 20.04,22.48 20.04,22.8 19.63,23.2 | v24.84,8.87 24.89,8.81 R7.1
  Top 0.381: C23.2 14.84,23.93 | 15.87,19.76 15.87,19.28 C1.2 | v17.52,20.32 18.07,19.77 R15.2 R18.2 | U6.29 51.8,25.34 v52.12,25.65 52.5,25.27 U6.30 | U6.13 40.6,22.39 v40.18,21.97 | C10.2 25.92,23.33 v25.89,23.36 | 21.46,21.34 21.31,21.19 v20.06,21.19 20.06,21.96 U5.8 | 51.99,12.7 51.51,12.7 | C4.2 64.74,29.63 64.78,29.59
  Top 0.508: C22.2 v14.16,25.19 | C23.2 14.87,23.95 v14.14,23.95 | v16.79,20.7 16.79,19.77 C1.2 | v64.69,36.83 64.82,36.7 64.82,29.55 64.78,29.59 64.78,5.17
  Top 0.61: C30.1 57.8,5.34 v58.44,4.7 | C30.1 v58.5,5.46 | C30.1 v57.8,6.21 v57.81,6.22
  Top 0.635: J2.3 63.32,12.47 v63.29,12.45 | J2.4 63.32,5.87 v63.16,5.71 | v56.89,34.16 56.87,34.18 U1.4 v55.75,35.43
  Bottom 0.254: D15.5 47.86,20.67 v48.69,20.67 | D15.10 46.07,20.66 v46.02,20.7 | R24.1 45.98,27.64 v46.02,27.69
  Bottom 0.305: R24.1 45.98,26.63
  Bottom 0.381: 46.2,15.95 v46.15,16 | D1.1 46.22,17.73
  Bottom 0.635: J3.6 51.67,24.45 52.12,24.89 v52.12,25.65
  other vias: 20.16,26.9 21.51,23.22 19.29,23.45 16.66,16.87 24.62,23.58 46.15,17.65 46.15,16.89 36.29,5.61 30.73,9.75 30.7,11.66 33.95,11.81 32.06,21.91 31.3,23.69 31.43,21.02 37.37,18.38 41.46,21.15 40.17,16.88 39.3,29.27 41.71,28.77 30.79,32.32 40.83,37.91 32.44,37.27 47.59,14.27 12.97,1.27 32.3,5.71 39.8,5.71 47.8,5.71 44.75,1.78 34.08,1.91 21.33,1.91 58.72,41.02 50.21,41.66 34.59,41.66 28.24,41.27 8.44,37.27 9.84,25.21 10.09,17.21 52.62,29.08 48.81,29.21 54.27,29.24 54.61,24.77 54.02,20.32 49.45,16.76 58.42,32.64 54.78,34.67 53.13,36.32 47.04,38.73 30.75,33.96 32.18,30.61 60.55,10.57 30.09,38.51 24.05,41.4 16.38,41.76 12.87,41.66 43.1,41.53 21.23,21.85 21.51,25.27 36.48,18.38 14.17,37.59 9.77,24.25 11.72,24.38 13.1,25.19 20.37,16.79 17.98,16.84 20.47,17.48 60.27,6.22 59.96,22.25 36.36,16.88 38.26,16.88 18.78,22.95 19.8,22.95 22.55,8.99 9.04,4.95 8.28,6.35 11.2,8.76 17.55,1.52 29.61,1.52 39.52,1.65 49.04,1.78 52.34,1.52 57.17,1.52 59.71,2.54 60.73,8.51 58.57,9.27 50.95,6.1 45.74,6.22 42.44,6.48 41.04,9.4 43.71,9.4 10.05,16.26 13.74,39.12 17.17,38.86 17.17,37.47 18.69,38.86 24.91,38.99 28.47,38.35 27.83,36.96 24.53,35.81 36.09,39.12 55.01,40.13 47.65,40.39 42.18,38.99 53.61,33.53 42.69,13.84 48.53,13.08 45.36,12.32 21.1,38.73 62.2,16.03 59.53,15.39 55.21,14.88 55.21,16.54 54.1,27.05 13.14,16.32 13.14,18.22 13.14,19.24 13.39,15.05 16.58,8.74 19.25,8.74
  pour Bottom (rank 6): 6.27,43.81 66.59,43.81 66.59,-0.64 6.27,-0.64
  pour Top (rank 6, no thermals): 6.27,43.81 66.59,43.81 66.59,-0.64 4.36,-0.64 4.36,0.64 6.27,0.64
  pour Top (no thermals): 21.76,17.65 20.75,17.65 20.37,18.03 18.46,18.03 18.46,17.53 18.21,17.27 16.68,17.27 16.43,17.02 16.43,16.64 16.56,16.51 19.35,16.51 19.48,16.64 20.49,16.64 20.87,17.02 21.76,17.02 21.89,17.14 21.89,17.53
IIC_ADDR  (via drill 0.25 pad 0.51)
  Top 0.152: v44.09,27.69 44.09,26.71 42.94,25.56 42.37,25.56 41.99,25.18 U6.15
  Bottom 0.152: JP1.MM 44.59,28.28 44.59,28.18 v44.09,27.69
INT  (via drill 0.25 pad 0.51)
  Top 0.152: v58.16,34.16 58.14,34.18 U1.3 | R2.1 62.25,35.03 v62.15,34.92
  Bottom 0.152: TP2.T 58.16,33.64 v58.16,34.16 58.92,34.92 v62.15,34.92
N$1
  pour Top (no thermals): 24.76,17.73 26.74,17.73 26.94,17.93 26.94,18.69 26.74,18.9 23.39,18.9 23.29,18.8 23.29,18.08 23.39,17.98 24.51,17.98
N$5  (via drill 0.25 pad 0.51, 0.35)
  Top 0.381: v39.29,20.57 v39.29,13.97 | v33.19,29.72 31.67,28.19 v31.67,26.04 | v57.21,28.84 57.21,28.12 D3.+
  Bottom 0.152: BAT1.V+@1 36.45,29.61
  Bottom 0.381: BAT1.V+@2 37.01,13.97 v39.29,13.97 | v31.67,26.04 31.54,25.91 31.54,25.09 32.13,24.51 38.53,24.51 39.29,23.75 v39.29,20.57 | BAT1.V+@1 35.72,29.72 v33.19,29.72 | 36.45,29.61 37.29,30.45 55.6,30.45 v57.21,28.84
N$6
  Top 0.152: R4.2 20.53,8.09 Q1.3
N$7
  Top 0.152: D5.+ 18.86,7.69 19.22,7.33 R4.1 19.84,5.35 19.98,5.21 20.11,5.08 20.69,4.51 BUZ1.-
N$8
  Top 0.152: Q1.1 22.94,7.52 R3.2 24.87,7.52 R7.2
N$9
  Top 0.152: C5.2 30.43,18.82 32.89,21.29 U6.2
N$10
  Top 0.152: U1.1 60.68,34.44 61.08,34.04 X1.2 63.63,34.04 63.82,33.85 63.82,31.62 63.62,31.42 C13.2
N$11
  Top 0.152: U1.2 59.41,33.8 60.8,32.41 X1.1
N$12
  Top 0.152: C6.2 31.82,14.96 31.42,15.37 31.42,18.16 34.29,21.04 U6.4
N$13
  Top 0.152: C5.1 30.93,14.99 30.93,18.57 33.59,21.22 U6.3
N$14
  Top 0.152: C6.1 31.85,15.53 31.85,17.84 34.99,20.97 U6.5
N$15
  Top 0.152: R22.1 51.51,17.62 49.7,19.44 49.7,19.81 49.69,19.82 U6.26
N$16
  Top 0.152: C8.2 52.6,17.55 50.4,19.75 50.4,20.45 U6.27
N$17
  Top 0.152: C9.2 53.93,17.36 51.1,20.19 51.1,20.45 U6.28
N$18
  Top 0.152: R23.2 33.04,18.26 35.69,20.91 U6.6
N$19
  Bottom 0.152: JP1.11 46.75,28.15 R24.2
N$20
  Bottom 0.152: JP1.00 43.48,28.44 43.48,27.43 43.82,27.09 R25.2
N$21
  Top 0.254: U3.4 23.87,24.76 23.71,24.92 23.71,25.71 R40.1 R41.2
N$22
  Top 0.305: R6.1 21.32,18.44 U4.1
  pour Top (no thermals): 17.32,19.3 21.51,19.3 22.02,18.8 22.02,18.29 21.76,18.03 21,18.03 20.62,18.41 17.32,18.41 17.19,18.54 17.19,19.18
N$23
  Top 0.381: C4.1 61.89,29.63 | 61.89,29.63 61.42,30.1 U1.8 60.68,28.42 61.5,29.23 | 61.5,29.23 61.5,28.57 D4.- D3.- | 61.89,29.63 61.5,29.23
N$24
  Top 0.305: R1.1 21.89,20.54 R6.2
N$26
  Top 0.305: U5.3 16.77,23.2 16.56,22.99 16.84,22.7 U5.4
  pour Top (no thermals): 17.47,23.32 16.2,23.32 15.84,22.96 15.84,21.79 15.95,21.69 16.61,21.69 17.47,22.56
N$27
  Top 0.152: U4.5 23.05,17.31 22.78,17.58 22.78,19.07 23.1,19.39 R11.1 R1.2
N$29
  pour Top (no thermals): 25.67,25.53 25.67,26.9 25.57,27 24.56,27 24.4,26.85 24.4,25.73 24.73,25.4 24.73,24.46 24.81,24.38 24.96,24.38 25.01,24.43 25.01,24.87
N$30
  Top 0.152: R17.1 22.85,23.07 23.27,23.49 23.27,24.91 21.74,26.44 21.74,34.77 23.67,36.7 23.67,38.86 22.91,39.62 16.85,39.62 16.77,39.71 16.47,40.01 D16.-
N$31
  Top 0.152: U5.9 22.07,22.7 R17.2
N$33
  Top 0.152: R18.1 19.35,20.54 | 19.35,20.54 19.55,20.54 | 19.55,20.54 19.71,20.54 | 19.71,20.54 R16.2 | 19.55,20.54 19.54,20.55 19.54,20.7 | U5.7 19.54,20.73 | 19.54,20.73 19.35,20.54 | 19.54,20.73 19.54,20.7 | 19.54,20.7 19.71,20.54
N$34
  Top 0.152: U5.11 21.95,23.7 R20.1
N$36
  Top 0.152: R19.1 21.47,24.6 21.08,24.2 U5.12
N$37
  Top 0.305: R15.1 18.27,21.43 18.54,21.69 U5.5
N$64
  Bottom 0.152: D15.14 D15.1 47.84,23.42 47.84,23.5 47.61,23.73 R60.1 47.7,23.86 48.43,24.59 48.43,26.16 48.92,26.65 J3.8
N$72
  Bottom 0.152: J3.1 48.66,18.95 47.95,19.66 D15.7 D15.8 46.59,18.84 R64.1
N$76
  Bottom 0.152: J3.7 49.34,25.55 48.94,25.15 48.94,23.88 48.48,23.41 48.48,22.41 48.23,22.16 D15.2 D15.13 46.21,22.16 45.64,22.73 R43.1
N$77
  Bottom 0.152: J3.5 50.32,23.37 49.32,23.37 48.99,23.03 48.99,22.04 48.61,21.66 D15.3 D15.12 46.04,21.66 45.85,21.85 R44.1
N$78
  Bottom 0.152: J3.3 D15.4 D15.11 46.38,21.16 46.22,21.31 45.69,21.31 45.39,21.01 R45.1
OLED_RST
  Top 0.152: D2.+ 34.55,14.38 C7.1 34.49,14.94 R21.1 34.49,17.43 38.4,21.34 40.28,21.34 41.29,22.34 | 41.29,22.34 41.3,22.35 41.3,22.48 U6.14 41.29,22.34
RESET
  Top 0.152: U2.15 11.73,19.6 11.73,7.24 14.88,4.09 K2.2
SWCLK  (via drill 0.25 pad 0.51)
  Top 0.152: v59.36,25.15 58.38,25.15 J7.1
  Bottom 0.152: U2.17 11.09,21.25 11.09,15.62 11.95,14.77 11.95,10.07 12.36,9.65 13.13,9.65 16.81,5.97 28.49,5.97 32.86,10.34 54.15,10.34 55.93,12.12 55.93,21.74 59.13,24.94 59.15,24.94 v59.36,25.15
SWDIO  (via drill 0.25 pad 0.51)
  Top 0.152: v59.36,24 58.97,24 58.21,23.24 J7.2
  Bottom 0.152: v59.36,24 56.38,21.03 56.38,11.89 54.4,9.91 32.94,9.91 28.62,5.59 16.68,5.59 13,9.27 12.24,9.27 11.6,9.91 11.6,14.61 10.71,15.49 10.71,19.09 U2.18
SYS_3V3  (via drill 0.25, 0.25 pad 0.51, 0.35)
  Top 0.152: 28.37,15.49 v28.49,15.37 | 63.91,30.51 64.12,30.72 64.12,30.86 | R2.2 63.83,35.03 64.12,34.74 64.12,30.86 | v63.94,30.48 63.94,30.67 64.12,30.86
  Top 0.254: 27.71,22.18 27.72,22.18 | R40.2 23.86,27.14 24.51,27.79 26.82,27.79 | 26.82,27.79 27.55,27.79 | 28.01,27.79 27.55,27.79 | 27.55,27.79 27.59,27.83 27.59,27.98 27.01,27.98 | 26.82,27.79 27.01,27.98 | 27.01,27.98 27.27,28.25 27.27,28.52
  Top 0.305: 28.24,7.72 28.29,7.67 | R10.2 R9.2 25.73,5.3 26.53,4.51 BUZ1.+
  Top 0.381: D4.+ v63.7,28.09 | R8.2 63.94,30.51 v63.94,30.48 | C24.2 42.34,8.64 | 42.34,8.64 C26.2 | 42.34,8.64 41.96,8.64 | 42.34,8.64 42.72,8.64 | C29.2 58.59,16.64 59.1,17.14 59.1,20.32 58.72,20.7 J7.3 | v41.6,33.68 41.75,33.53 C21.2 C20.2 41.76,34.16 v41.6,34.31
  Top 0.508: v30.73,12.49 30.73,13.14 FB1.1 30.74,13.13 v31.36,13.13
  Top 0.559: v28.29,8.79 28.24,8.84 27.68,8.84 v27.66,8.81 28.12,8.35 | 28.12,8.35 28.24,8.23 28.24,7.24 | 28.12,6.96 28.12,8.35 | 28.29,7.67 28.78,7.19 29.05,7.19
  Top 0.635: v28.49,15.37 28.49,20.57 | v27.61,21.46 28.01,21.06 | 28.01,21.06 28.49,20.57 | U2.12 J11.3 | 28.53,22.18 27.71,22.18 | 28.01,27.79 27.27,28.52 27.22,28.57 v27.22,34.29 | 28.09,27.71 29,26.8 29,23.42 | 29,23.42 29,22.66 28.53,22.18 | J6.3 45.7,7.37 44.37,7.37 43.1,8.64 42.72,8.64 | 28.34,7.19 28.12,6.96 28.12,6.22 28.12,5.72 27.29,4.89 27.22,4.83 26.91,4.51 BUZ1.+ 26.71,3.55 26.21,3.05 20.87,3.05 16.27,7.65 D5.- | 28.34,7.19 29.05,7.19 33.92,7.19 J5.3 37.15,7.19 40.25,7.19 41.7,8.64 41.96,8.64 | J7.3 56.76,20.7 55.41,22.06 55.41,27.18 | 55.41,27.18 55.41,27.7 | 55.41,27.7 55.41,29.74 54.68,30.47 52.47,30.47 J1.3 | 28.01,21.06 28.01,21.39 | 28.01,21.39 28.01,21.67 28.53,22.18 | 28.01,21.39 28.49,21.87 | 28.49,21.87 28.65,22.02 29.2,22.02 28.49,21.31 | 28.49,21.87 28.49,21.31 | 28.49,21.31 28.49,20.57 | C10.1 28.16,22.94 28.52,22.94 29,23.42 | 28.34,7.19 28.24,7.19 28.24,7.24 28.24,7.72 | v28.29,8.79 28.29,7.67 | D4.+ 62.62,27.52 62.28,27.18 55.93,27.18 | 55.93,27.18 55.41,27.18 | 55.41,27.7 55.93,27.18 | 55.93,27.18 55.42,26.67
  Bottom 0.305: v27.6,21.46 v27.61,21.46 | 28.93,12.49 28.75,12.49 | 28.75,12.49 28.31,12.49 | 28.31,12.49 28.24,12.42 | v31.36,13.13 31.12,12.89 | 31.12,12.89 31.02,12.79 | 31.02,12.79 v30.73,12.49 | 28.63,13.13 28.4,13.13 28.25,12.98 | 28.24,12.97 28.42,12.79 | 31.02,12.79 28.77,12.79 | 28.77,12.79 28.42,12.79 | 28.42,12.79 28.52,12.89 31.12,12.89 | 28.77,12.79 28.24,12.25 28.24,11.99 | 28.75,12.49 28.24,11.99 | 28.24,11.99 28.24,11.81 | 28.31,12.49 28.25,12.55 28.25,13.51
  Bottom 0.381: v63.7,28.09 63.7,29.92 63.94,30.16 v63.94,30.48
  Bottom 0.559: 27.78,9.27 27.66,9.14 v27.66,8.81
  Bottom 0.635: 28.7,15.52 42.82,15.52 43.29,15.06 FB3.1 46.79,15.04 | v28.49,15.37 28.55,15.37 28.7,15.52 | 27.67,21.53 v27.6,21.46 | J1.3 49.14,34.31 47.94,35.51 38.16,35.51 37.54,34.89 | J4.3 37.54,34.89 | 37.54,34.89 36.82,35.61 36.55,35.61 | v28.49,15.37 28.25,15.13 28.25,13.87 | 28.25,13.51 28.25,12.98 28.24,12.97 28.24,12.42 28.24,11.81 28.29,11.76 v28.29,8.79 27.78,9.3 | 28.25,13.51 28.25,13.87 | v27.78,15.37 v28.49,15.37 | v27.78,15.37 27.78,13.26 | 27.78,13.26 27.78,11.58 | 27.78,11.58 27.78,9.3 | 27.78,9.27 27.78,9.3 | 28.7,15.52 27.94,15.52 v27.78,15.37 | v31.36,13.13 30.77,12.54 30.7,12.54 31.3,13.13 v31.36,13.13 | v31.36,13.13 28.63,13.13 28.25,13.51 | v30.73,12.49 29.23,12.49 | 29.23,12.49 28.93,12.49 | 28.93,12.49 28.55,12.49 27.78,13.26 | 28.93,12.49 28.01,11.58 27.78,11.58 | 28.25,13.87 29.23,12.89 29.23,12.49
  Bottom 0.762: 28.55,34.29 v27.22,34.29 18.03,34.29 J11.3
  other vias: 27.88,34.29
  pour Top (no thermals): 26.56,27.13 27.27,27.13 28.14,26.26 28.14,21.97 28.01,21.84 27.33,21.84 27.17,22 27.17,25.25 27,25.43 26.41,25.43 26.28,25.55 26.28,26.85
  pour Top (no thermals): 27.07,34.82 28.19,34.82 28.37,34.65 28.37,29.87 29.79,28.45 29.79,22.23 29.1,21.54 27.81,21.54 27.68,21.67 27.68,22.33 28.49,23.14 28.49,26.34 26.87,27.97 26.87,34.62
  pour Bottom (no thermals): 14.85,32.18 17.88,35.2 29.51,35.2 30.45,36.14 49.12,36.14 49.96,35.31 49.96,33.22 49.78,33.05 49.4,33.05 47.26,35.18 44.24,35.18 42.46,33.4 41.19,33.4 40.81,33.78 40.81,34.92 40.56,35.18 30.88,35.18 29.61,33.91 18.46,33.91 15.74,31.19 15.29,31.19 14.85,31.62
  pour Top: 27.22,22.89 27.22,15.16 27.5,14.88 28.67,14.88 28.77,14.99 28.77,22.83 28.49,23.11 27.45,23.11
USB_5V  (via drill 0.25 pad 0.51)
  Top 0.305: v20.54,19.89 20.42,19.77 R16.1
  Bottom 0.305: v20.54,19.89 19.3,19.89 19.17,19.76 17.32,19.76 16.81,19.76 16.67,19.9 16.15,20.42 16.15,21.23 16.15,23.39 v16.58,23.82
  pour Top (no thermals): 11.67,32.9 9.78,32.9 9.49,32.61 9.49,27.66 11.33,25.82 15.39,25.82 15.54,25.67 15.54,23.83 15.79,23.57 17.99,23.57 18.01,23.6 18.01,23.79 17.95,23.85 17.29,23.85 16.44,24.7 16.44,26.2 15.67,26.97 13.39,26.97 12.02,28.33 12.02,32.55
VBAT
  Top 0.254: 18.38,26.36 18.13,26.36 18.13,26.11 | 18.38,26.36 18.56,26.36 | 18.56,26.36 18.67,26.36 | 18.3,25.55 18.13,25.72 18.13,25.91 | 18.13,25.91 18.13,25.96 | 18.13,25.96 18.13,26.11 | 18.13,26.11 18.38,26.36 | 18.47,26.25 18.13,25.91 | 18.47,26.25 18.56,26.34 18.56,26.36 | 18.13,25.96 18.3,25.79 18.3,25.55 | 18.47,26.17 18.36,26.05 18.36,25.91 18.36,25.6 18.3,25.55 | 18.47,26.17 18.47,26.25 | 18.47,26.25 18.56,26.25 | 18.56,26.25 18.67,26.36 | 18.67,26.36 18.7,26.39 18.92,26.39 19.15,26.39 19.27,26.26 | 18.56,26.25 18.47,26.17 | 16.67,26.9 16.63,26.9 16.2,27.33
  Top 0.305: 14.4,32.89 14.4,28.35 15.16,27.58 16.33,27.58 16.89,27.03 17.36,26.56 17.56,26.56 | C25.1 18.12,25.99 17.74,26.37 | 17.74,26.37 17.56,26.56 | 18.13,26.11 18.03,26.21 17.55,26.21 17.33,26.43 | 18.13,25.91 17.74,26.3 17.74,26.37 | 17.56,26.56 18.98,26.56 19.27,26.26 19.48,26.06 19.54,26 19.54,25.5 U5.14 | 18.13,25.72 17.42,26.43 17.33,26.43 | 17.33,26.24 17.63,25.94 U5.16 18.54,25.31 18.3,25.55 | 17.33,26.24 17.33,26.43 | 17.33,26.24 16.67,26.9
  Top 0.33: 18.54,25.31 18.58,25.35 18.58,25.45 18.68,25.55 | 19.54,25.5 19.26,25.78 18.92,25.78 | 19.48,26.06 19.17,26.06 | 19.17,26.06 18.92,26.06 | 18.92,26.06 18.74,26.06 | 18.74,26.06 18.51,26.06 18.36,25.91 | 18.92,25.78 18.77,25.63 | 18.3,25.55 18.68,25.55 | 18.68,25.55 18.77,25.63 | 18.36,25.6 18.38,25.63 18.77,25.63 | 18.3,25.79 18.91,25.79 18.92,25.78 | 18.92,26.06 18.92,26.39 19.17,26.14 19.17,26.06 | 18.67,26.36 18.67,26.13 18.74,26.06 | 16.67,26.9 16.67,27.27 | 16.67,27.27 16.64,27.3 16.64,27.77 16.68,27.81 | 16.68,27.81 16.68,26.82 16.94,27.07 16.94,27.41 | 16.68,27.81 16.68,33.57 16.57,33.57 16.35,33.35 16.25,33.25 | 16.68,33.4 16.68,33.25 16.28,33.25 | 16.89,27.03 16.89,27.06 16.67,27.27 | 16.94,27.41 16.94,28.25 | 16.94,28.25 16.94,32.59 | 16.94,32.59 16.94,34.24 17.04,34.34 | 16.33,27.58 16.33,27.64 16.94,28.25 | 15.97,27.33 17.36,25.94 17.63,25.94 | 16.94,27.41 18.35,25.99 C25.1 | 14.75,33.25 14.4,32.89 | 16.25,33.25 15.23,33.25 | 16.25,33.25 16.28,33.25 | 16.28,33.25 16.94,32.59
  Top 0.381: 16.2,27.33 15.97,27.33 15.11,27.33 14.19,28.25 14.19,32.94 14.8,33.55 15.03,33.55
  Top 0.635: 16.54,33.85 15.32,33.85 15.03,33.55 15.23,33.35 16.35,33.35 | 15.23,33.25 14.75,33.25
  Top 0.889: 16.54,33.85 16.54,33.9 18.59,35.94 21,35.94 SW1.COM2
  Bottom 0.889: SW1.COM2 SW1.COM1
VBOOST_5V  (via drill 0.25 pad 0.51, 0.38 pad 0.51)
  Top 0.305: R5.1 17.63,17.83 14.83,17.83 14.52,17.53 | 14.27,9.93 14.93,9.27 15.01,9.27
  Top 0.381: 15.01,9.27 16.28,9.27 16.76,9.75 16.76,14.15 15.92,14.99 14.65,14.99 | 14.93,9.27 14.68,9.02 14.27,9.02
  Top 0.559: 14.27,9.93 14.27,14.99 14.4,14.99 14.65,14.99
  Top 0.635: C28.1 60.4,16.48 60.37,16.51 v60.37,16.89
  Top 0.889: J7.6 v61.39,20.7 | 14.27,9.93 14.27,9.02 14.27,6.58 v14.19,6.5 | 14.4,14.99 14.4,16.89 v14.52,17.02 14.52,17.53 | v14.96,5.99 14.75,5.99 14.27,6.48
  Bottom 0.635: 14.22,17.58 v14.52,17.58 v14.52,17.02
  Bottom 0.889: 58.34,16.89 58.34,11.02 51.76,4.45 17.83,4.45 17.27,4.45 16.17,4.45 | v60.37,16.89 59.1,16.89 | 59.1,16.89 58.34,16.89 | 58.34,16.89 58.34,17.66 | 58.34,17.66 58.34,19.3 59.74,20.7 v61.39,20.7 | 58.34,17.66 59.1,16.89 | 59.1,16.89 58.34,16.13 | 14.19,6.46 14.21,6.48
  pour Top (no thermals): 17.95,18.16 14.17,18.16 13.89,17.88 13.89,16.92 14.17,16.64 14.65,16.64 15.54,17.53 17.83,17.53 17.95,17.65
  pour Bottom (isolate 0.152, no thermals): 14.27,6.86 14.52,6.86 16.56,4.83 16.56,4.32 16.17,3.94 15.79,3.94 13.38,6.35 13.38,6.6 13.63,6.86
VDD_3V3_OLED  (via drill 0.25 pad 0.51)
  Top 0.305: R21.2 33.73,16.61 | R23.1 32.27,16.61 v32.43,16.76 | D2.- 32.3,13.73 | U6.9 37.8,22.32 | 37.8,22.32 38.02,22.1 | 38.02,22.1 38.91,22.1 39.2,22.39 U6.11 39.2,25.44 39.92,26.16 v42.72,26.16 | 37.8,22.32 37.8,21.88 | 37.8,21.88 33.73,17.8 33.73,16.92 | 37.8,21.88 38.02,22.1 | 33.73,16.92 33.73,16.61 | 33.73,16.61 v33.57,16.76 33.73,16.92
  Top 0.381: D2.- 32.23,13.02 32.56,12.7 34.84,12.7 35.35,13.21 v35.35,16.76
  Top 0.508: FB1.2 31.85,14.04 D2.-
  Bottom 0.305: R25.1 45.33,26.62 44.88,26.16 v42.72,26.16
  Bottom 0.381: v35.35,16.76 v33.57,16.76 v32.43,16.76
VDD_3V3_SD  (via drill 0.25 pad 0.51)
  Top 0.305: v44.12,18.29 44.24,18.41 v48.18,18.41 | v46.91,25.91 47.42,26.42 47.8,26.42 51.61,26.42 51.99,26.42 52.62,26.42 53.26,25.78 53.26,24.38 53.26,22.35 52.75,21.84 52.24,21.84 v51.61,21.84
  Bottom 0.254: R63.2 44.54,19.28 45.34,20.08 R62.2 | 46.84,23.87 R60.2 45.68,23.86 R61.2
  Bottom 0.305: R63.2 44.54,18.71 v44.12,18.29 | v48.18,18.41 47.79,18.41 R64.2 | v46.91,25.91 46.85,25.85 R60.2
  Bottom 0.381: R64.2 47.6,18.56 47.6,18.03 | 47.6,18.03 D1.2 | D1.2 47.6,17.4 | 47.6,17.4 C2.1 C3.1 47.6,15.12 FB3.2 | D1.2 47.91,17.73 | 47.93,17.73 48.81,17.73 51.05,17.73 51.42,18.1 51.61,18.29 51.61,20.95 v51.61,21.84 51.2,22.25 J3.4 | 47.6,18.03 47.91,17.73 | 47.91,17.73 47.93,17.73 | 47.93,17.73 47.6,17.4
VSYS  (via drill 0.25, 0.25 pad 0.51)
  Top 0.152: 14.23,22.72 11.55,25.4 11.15,25.4 9.08,27.47 9.08,32.88 9.75,33.55 13.23,33.55 15.71,36.03 D16.+
  Top 0.254: 17.6,24.2 U5.1 18.66,24.2 19.04,24.58 U5.15 | U3.5 23.87,22.43 v23.49,22.05
  Top 0.305: C14.1 16.81,15.69 | C16.2 19.39,15.71 C18.1 | U3.7 24.87,21.68 C15.2 25.37,21.66 U3.8
  Bottom 0.305: v23.49,22.05 23.49,20.83 24.28,20.04 | v25.09,19.61 24.71,19.61 24.28,20.04 | 24.28,20.04 24.28,19.28 | 24.28,20.04 25.04,20.04
  other vias: 14.98,19.71 14.27,19.08 14.27,19.68 17.11,24.66 16.89,25.17 25.98,19.63 17.62,24.87 25.98,20.32 17.06,14.94 16.53,15.85 16.62,15.3
  pour Top (no thermals): 15.08,22.96 14.14,22.96 14.02,22.83 14.02,18.97 14.3,18.69 14.88,18.69 15.24,19.05 15.24,22.81
  pour Bottom (no thermals): 17.55,25.5 16.25,25.5 14.57,23.83 14.57,21.44 13.99,20.85 13.99,19 14.59,18.4 15.79,19.61 15.79,23.57 16.56,24.33 17.62,24.33 17.78,24.49 17.78,25.27
  pour Top (no thermals): 24.79,22.38 24.79,19.56 25.01,19.33 26.08,19.33 26.26,19.51 26.26,21.36 25.24,22.38
  pour Bottom (no thermals): 13.99,20.45 13.99,18.64 14.44,18.2 15.27,18.2 15.83,17.64 15.83,15.23 16.37,14.69 17.25,14.69 17.38,14.82 17.38,17.66 17.67,17.96 24.71,17.96 26.26,19.51 26.26,20.42 26.11,20.57 25.14,20.57 23.9,19.33 16.84,19.33 15.62,20.55 14.09,20.55
  pour Top (no thermals): 20.47,16.1 15.93,16.1 15.67,15.84 15.67,15.36 16.32,14.71 20.75,14.71 21.51,15.47 26.34,15.47 26.92,16.05 26.92,16.97 26.74,17.14 25.62,17.14 25.14,16.66 21.03,16.66
  pour Top (no thermals): 16.76,25.45 17.6,25.45 17.8,25.25 17.8,24.08 17.32,24.08 16.63,24.77 16.63,25.32

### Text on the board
tNames: IIC | IIC | ON | OFF | USB5V | G | 3V3 | 10 | 9 | 8 | 7 | SCL | · | 5 | SDA | · | 4 | 3V3 | GND | SCL | · | 5 | SDA | · | 4 | 3V3 | GND | 7 | 1 | 30 | SWCLK | · | RX | GND | 6 | · | SWCLK | SWDIO | TX | 3V3 | 5V | SWDIO | GND | GND | - | RESET | GND | 3V3 | N/A | 0 | GND | 3V3 | TX | · | 6 | RX | · | 7 | 0 | 1 | 2 | 3 | 4 | 5 | 6 | Buzzer(A3) | + | RESET | Button(D1) | A0 | · | D0 | UART
bNames: ·
tTest: JP3
Reference: JP3 | JP4 | JP5 | JP6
